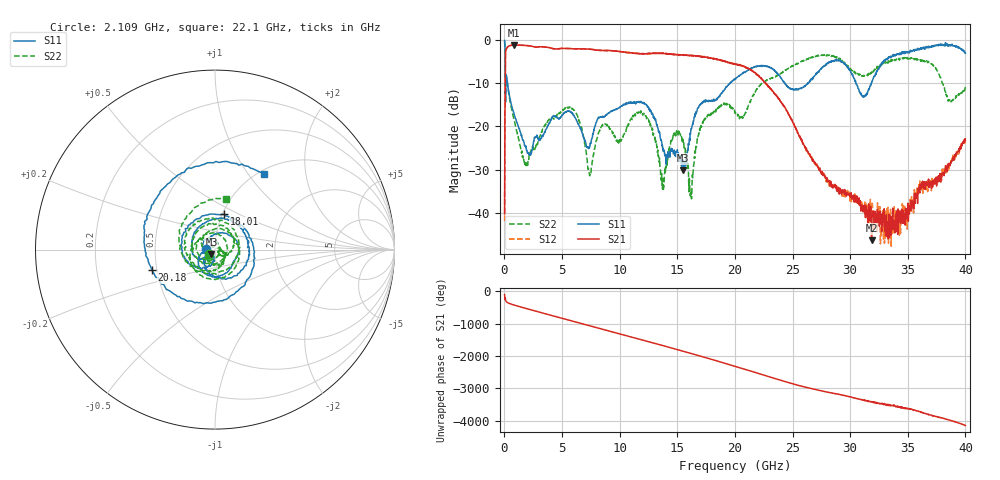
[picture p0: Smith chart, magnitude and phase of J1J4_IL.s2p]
!Agilent Technologies,N5230A,US43500312,A.07.50.67
!Agilent N5230A: A.07.50.67
!Date: Thursday, March 05, 2015 11:25:03
!Correction: S11(Full 2 Port(1,2))
!S21(Full 2 Port(1,2))
!S12(Full 2 Port(1,2))
!S22(Full 2 Port(1,2))
!S2P File: Measurements: S11, S21, S12, S22:
# Hz S  dB  R 50
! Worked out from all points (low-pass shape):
!   1601 points, 10 MHz to 40 GHz, reference 50 ohm
!   highest |S21| = -1.17 dB at 834.8 MHz (marker M1); lowest = -46.3 dB at 31.85 GHz (marker M2)
!   |S21| within 3 dB of the highest: 82.76 MHz to 17.83 GHz (17.74 GHz wide, 198 % of centre); 17.89092 GHz to 17.92791 GHz (36.99 MHz wide, 0.207 % of centre)
!   lowest |S11| = -30.1 dB at 15.51 GHz (marker M3), VSWR 1.06, Z = 48 - j2.29 ohm
!   |S11| at or under -10 dB: 258.4 MHz to 19.55 GHz (19.29 GHz wide, 195 % of centre); 24.32 GHz to 26.3 GHz (1.986 GHz wide, 7.84 % of centre); 30.5 GHz to 31.83 GHz (1.33 GHz wide, 4.27 % of centre)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
!   |S22| runs from -36.7 to -0.2 dB; largest |S21 - S12| = 0.019
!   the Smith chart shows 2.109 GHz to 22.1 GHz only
!   S11 on the Smith chart (normalised r, x): 2.109 GHz: 0.91, +0.01; 18.01 GHz: 1.02, +0.42; 20.18 GHz: 0.47, -0.12; 22.1 GHz: 1.06, +1.20
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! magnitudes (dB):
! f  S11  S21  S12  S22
! 10 MHz  -0.1  -40.2  -41.9  -0.2
! 259.9 MHz  -10.0  -1.7  -1.7  -10.3
! 834.8 MHz  -17.1  -1.2  -1.2  -18.4
! 2.109 GHz  -26.4  -1.4  -1.3  -27.6
! 5.234 GHz  -16.7  -2.0  -2.0  -16.0
! 6.683 GHz  -21.1  -2.1  -2.1  -20.2
! 7.383 GHz  -24.8  -2.1  -2.1  -31.3
! 8.508 GHz  -17.8  -2.4  -2.5  -19.5
! 11.63 GHz  -14.3  -3.1  -3.2  -16.8
! 13.36 GHz  -21.1  -3.1  -3.1  -26.7
! 13.76 GHz  -25.0  -3.2  -3.1  -32.0
! 15.51 GHz  -30.1  -3.5  -3.5  -23.2
! 16.18 GHz  -20.8  -3.6  -3.6  -35.7
! 16.93 GHz  -15.0  -3.8  -3.9  -20.6
! 18.01 GHz  -13.9  -4.3  -4.2  -16.9
! 20 GHz  -9.0  -5.6  -5.6  -16.6
! 20.18 GHz  -8.6  -5.7  -5.8  -17.2
! 22.1 GHz  -6.0  -8.4  -8.5  -10.7
! 26.68 GHz  -9.1  -27.5  -27.6  -4.1
! 31.85 GHz  -10.0  -46.3  -37.8  -7.5
! 33.35 GHz  -3.9  -41.2  -40.9  -5.1
! 40 GHz  -3.1  -23.1  -23.1  -10.9
